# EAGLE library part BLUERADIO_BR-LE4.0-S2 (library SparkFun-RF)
Blue Radios BR-LE4.0-S2A BlueTooth 4.0 Module The BR-LE4.0-S2A is a standalone Class 1 Bluetooth 4.0 module that requires no firmware or external components. Custom client applications can be written directly onto the module, which supports both analog and digital peripherals, eliminating the need for a second microprocessor. Alternately, the BR-LE4.0-S2A can be integrated into an existing design as a HCI network processor device, with a host processor running the core application and the BR-LE4.0-S2A providing Bluetooth low energy communications. SparkFun Products: Bluetooth 4.0 Module - BR-LE 4.0-S2A (WRL-12991)
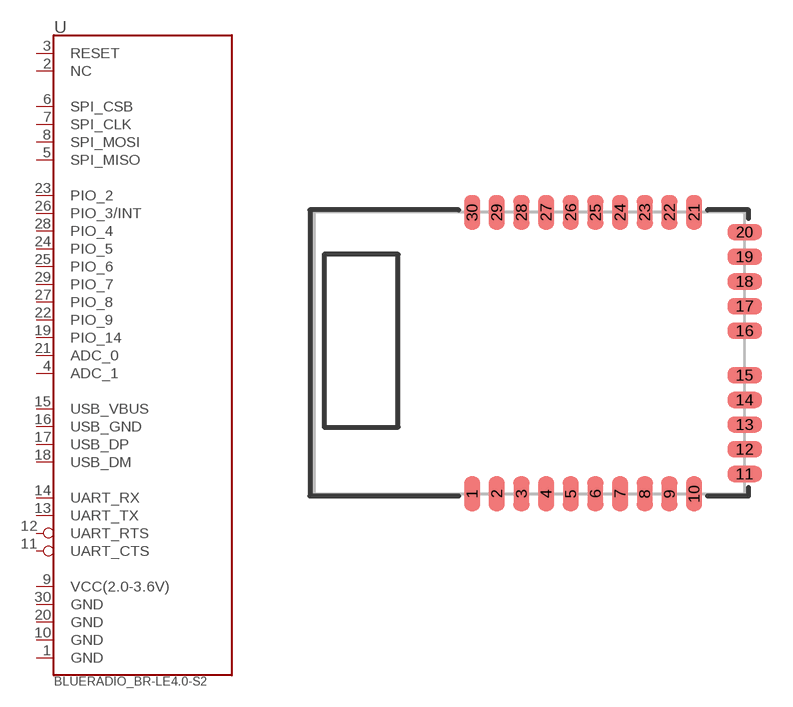
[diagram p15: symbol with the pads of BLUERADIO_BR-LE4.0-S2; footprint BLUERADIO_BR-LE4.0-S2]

Designator prefix -

## BLUERADIO_BR-LE4.0-S2 (PROD_ID: IC-11328; VALUE: BR-LE4.0-S2A)  [BLUERADIO_BR-LE4.0-S2]
1  GND  pwr
2  NC  nc
3  RESET  in
4  ADC_1  in
5  SPI_MISO
6  SPI_CSB
7  SPI_CLK
8  SPI_MOSI
9  VCC(2.0-3.6V)  pwr
10  GND  pwr
11  UART_CTS  in
12  UART_RTS  out
13  UART_TX  out
14  UART_RX  in
15  USB_VBUS
16  USB_GND
17  USB_DP
18  USB_DM
19  PIO_14
20  GND  pwr
21  ADC_0  in
22  PIO_9
23  PIO_2
24  PIO_5
25  PIO_6
26  PIO_3/INT
27  PIO_8
28  PIO_4
29  PIO_7
30  GND  pwr

## Footprint BLUERADIO_BR-LE4.0-S2 (pad centres in mm)
BlueRadio BR-LE4.0-S2 Bluetooth 4.0 Module 11.8x17.6x1.9mm Datasheet
smd 0.65 x 1.4: 1 -4.5,-5.7; 2 -3.5,-5.7; 3 -2.5,-5.7; 4 -1.5,-5.7; 5 -0.5,-5.7; 6 0.5,-5.7; 7 1.5,-5.7; 8 2.5,-5.7; 9 3.5,-5.7; 10 4.5,-5.7; 21 4.5,5.7; 22 3.5,5.7; 23 2.5,5.7; 24 1.5,5.7; 25 0.5,5.7; 26 -0.5,5.7; 27 -1.5,5.7; 28 -2.5,5.7; 29 -3.5,5.7; 30 -4.5,5.7
smd 1.4 x 0.65: 11 6.55,-4.9; 12 6.55,-3.9; 13 6.55,-2.9; 14 6.55,-1.9; 15 6.55,-0.9; 16 6.55,0.9; 17 6.55,1.9; 18 6.55,2.9; 19 6.55,3.9; 20 6.55,4.9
